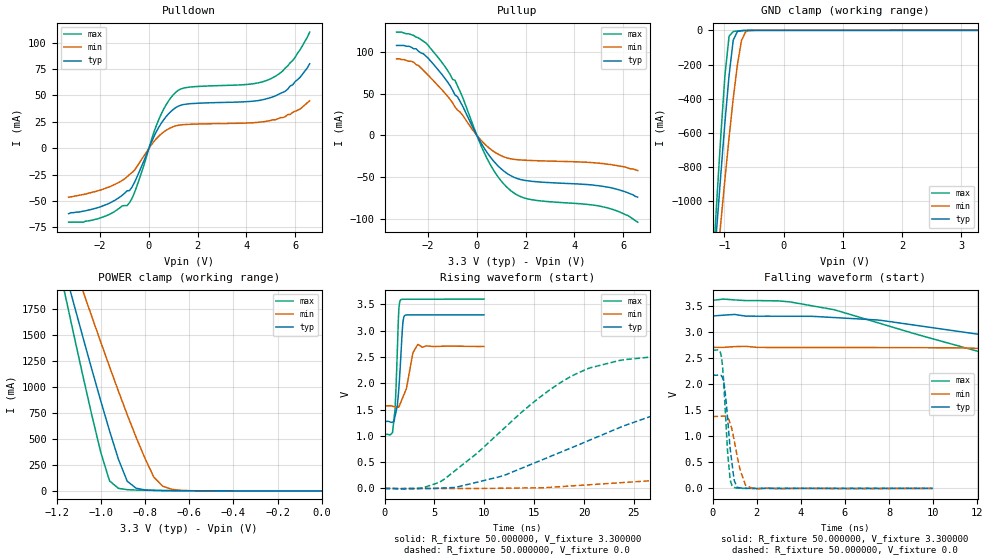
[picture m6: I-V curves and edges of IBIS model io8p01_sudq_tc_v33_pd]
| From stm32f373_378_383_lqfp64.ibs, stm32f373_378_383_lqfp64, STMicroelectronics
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|   Model io8p01_sudq_tc_v33_pd
[Model]  io8p01_sudq_tc_v33_pd
Model_type I/O
Polarity   Non-Inverting
Enable   Active-Low
Vinl =   0.990000V
Vinh =   2.310000V
Vmeas =  1.650000V
Cref =   50.000000pF
Rref =   100.000000M
Vref =   0.0V
C_comp   1.325200pF   1.251200pF   1.426700pF
[Temperature Range]   25.000000   0.125000k   -40.000000
[Pullup Reference]   3.300000V   2.700000V   3.600000V
[Pulldown Reference]   0.0V   0.0V   0.0V
[POWER Clamp Reference]   3.300000V   2.700000V   3.600000V
[GND Clamp Reference]   0.0V   0.0V   0.0V
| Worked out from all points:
|   slope of the pulldown table from 0 to 0.495 V, typ, clamps not added: 21.3 ohm
|   slope of the pullup table from 0 to 0.495 V, typ, clamps not added: 20.9 ohm
|   GND clamp passes 1 mA (typ) near -0.66 V on its own axis
|   POWER clamp passes 1 mA (typ) near -0.60 V on its own axis
|   rising waveform, R_fixture 50.000000, V_fixture 3.300000: 20-80 % time 413ps typ, 774ps min, 302ps max; typ from 1.27 V to 3.3 V
|   rising waveform, R_fixture 50.000000, V_fixture 0.0: 20-80 % time 18.6ns typ, 46.7ns min, 10.2ns max; typ from 0 V to 2.17 V
|   falling waveform, R_fixture 50.000000, V_fixture 3.300000: 20-80 % time 26.4ns typ, 44.8ns min, 16.4ns max; typ from 3.3 V to 1.27 V
|   falling waveform, R_fixture 50.000000, V_fixture 0.0: 20-80 % time 298ps typ, 421ps min, 225ps max; typ from 2.17 V to 0 V
[Pulldown]
|Voltage   I(typ)   I(min)   I(max)
-3.3V     -62mA      -46.4mA    -70mA
-2.1V     -56.2mA    -40.3mA    -66.8mA
-800mV    -40.04mA   -24.9mA    -51.58mA
-500mV    -27.57mA   -17.6mA    -36.07mA
400mV     19.71mA    11.36mA    27.01mA
700mV     29.83mA    16.93mA    40.97mA
1.1V      38.46mA    21.2mA     53.02mA
1.6V      41.98mA    22.62mA    57.7mA
4.1V      44.26mA    24mA       60.59mA
5V        48mA       26.3mA     65.8mA
5.9V      60mA       34mA       83mA
6.6V      80mA       45mA       110mA
[Pullup]
|Voltage   I(typ)   I(min)   I(max)
-3.3V     108mA      92mA       124mA
-2.6V     104mA      88mA       120mA
-2.2V     98mA       78.2mA     113mA
-1.4V     71.8mA     53.6mA     86.1mA
-900mV    48.51mA    34.23mA    66.14mA
-700mV    41.33mA    28.36mA    53.31mA
400mV     -19.77mA   -12.52mA   -26.8mA
900mV     -37.48mA   -22.89mA   -50.99mA
1.4V      -48.39mA   -28.06mA   -66.43mA
2.2V      -54.79mA   -29.98mA   -76.75mA
5.3V      -61.7mA    -34.2mA    -86.4mA
6.6V      -74mA      -42mA      -104mA
[GND_clamp]
|Voltage   I(typ)   I(min)   I(max)
-3.3V     -9.739A    -9.975A    -9.587A
-1.2V     -1.489A    -1.65A     -1.416A
-1.13V    -1.162A    -1.385A    -1.009A
-1.06V    -842.3mA   -1.125A    -616.9mA
-990mV    -537.1mA   -870.2mA   -263mA
-920mV    -262.5mA   -625.3mA   -33.98mA
-850mV    -56.96mA   -397.5mA   -7.097mA
-780mV    -7.026mA   -202.3mA   -3.727mA
-710mV    -1.792mA   -58.24mA   -1.753mA
-640mV    -564.1uA   -8.795mA   -558.4uA
-570mV    -123.3uA   -1.303mA   -102.2uA
3.28V     84.11uA    64.12uA    93.81uA
[POWER_clamp]
|Voltage   I(typ)   I(min)   I(max)
-3.28V    9.897A     9.838A     9.594A
-1.16V    2.103A     2.419A     1.88A
-1.12V    1.788A     2.17A      1.488A
-1.08V    1.476A     1.923A     1.102A
-1V       868.1mA    1.435A     373.1mA
-960mV    578.2mA    1.196A     96.06mA
-880mV    93.24mA    734.1mA    12.01mA
-840mV    26.3mA     517.4mA    8.56mA
-760mV    5.106mA    134mA      5.119mA
-720mV    3.355mA    46.34mA    3.808mA
-600mV    1.005mA    2.564mA    1.072mA
0V        0A         0A         0A
[Ramp]
| variable   typ   min   max
dV/dt_r  1.29954/18.58866n   0.82686/46.65085n   1.58814/10.22225n
dV/dt_f  1.21518/26.34936n   0.67806/44.55462n   1.54236/16.35641n
R_load = 50.000000
[Rising Waveform]
R_fixture= 50.000000
V_fixture= 3.300000
V_fixture_min= 2.700000
V_fixture_max= 3.600000
|time   V(typ)   V(min)   V(max)
0s        1.274V     1.569V     1.029V
820.8ps   1.263V     1.562V     1.094V
1.061ns   1.375V     1.549V     1.533V
1.281ns   1.567V     1.546V     2.6V
1.441ns   1.915V     1.55V      3.415V
1.602ns   2.4V       1.624V     3.579V
1.942ns   3.262V     1.781V     3.596V
2.843ns   3.298V     2.575V     3.596V
3.323ns   3.298V     2.735V     3.596V
9.97ns    3.299V     2.699V     3.599V
[Rising Waveform]
R_fixture= 50.000000
V_fixture= 0.0
V_fixture_min= 0.0
V_fixture_max= 0.0
|time   V(typ)   V(min)   V(max)
0s        1.008nV    9.499nV    1.541nV
5.506ns   6.074mV    -223.1uV   116.9mV
12.01ns   249.7mV    4.956mV    1.148V
20.02ns   874.6mV    64.07mV    2.247V
30.03ns   1.584V     202.5mV    2.56V
37.54ns   1.897V     361.3mV    2.602V
48.05ns   2.064V     583.6mV    2.635V
69.07ns   2.143V     971.6mV    2.648V
107.6ns   2.166V     1.294V     2.647V
249.2ns   2.166V     1.377V     2.647V
[Falling Waveform]
R_fixture= 50.000000
V_fixture= 3.300000
V_fixture_min= 2.700000
V_fixture_max= 3.600000
|time   V(typ)   V(min)   V(max)
0s        3.299V     2.699V     3.599V
3.003ns   3.296V     2.697V     3.588V
5.506ns   3.27V      2.697V     3.42V
14.51ns   2.799V     2.647V     2.331V
21.02ns   2.397V     2.557V     1.763V
29.03ns   2.013V     2.396V     1.324V
38.04ns   1.712V     2.216V     1.128V
60.06ns   1.363V     1.893V     1.04V
88.09ns   1.288V     1.68V      1.029V
249.2ns   1.274V     1.569V     1.029V
[Falling Waveform]
R_fixture= 50.000000
V_fixture= 0.0
V_fixture_min= 0.0
V_fixture_max= 0.0
|time   V(typ)   V(min)   V(max)
0s        2.166V     1.377V     2.647V
400.4ps   2.155V     1.381V     2.526V
540.5ps   1.952V     1.384V     1.772V
700.7ps   1.25V      1.341V     605.8mV
800.8ps   755.5mV    1.24V      163.1mV
940.9ps   284.2mV    1.006V     26.15mV
1.101ns   30.82mV    653.2mV    5.925mV
1.502ns   1.535mV    56.4mV     113uV
1.902ns   -16.72uV   -14.42mV   30.39uV
9.97ns    1.008nV    9.499nV    1.541nV
